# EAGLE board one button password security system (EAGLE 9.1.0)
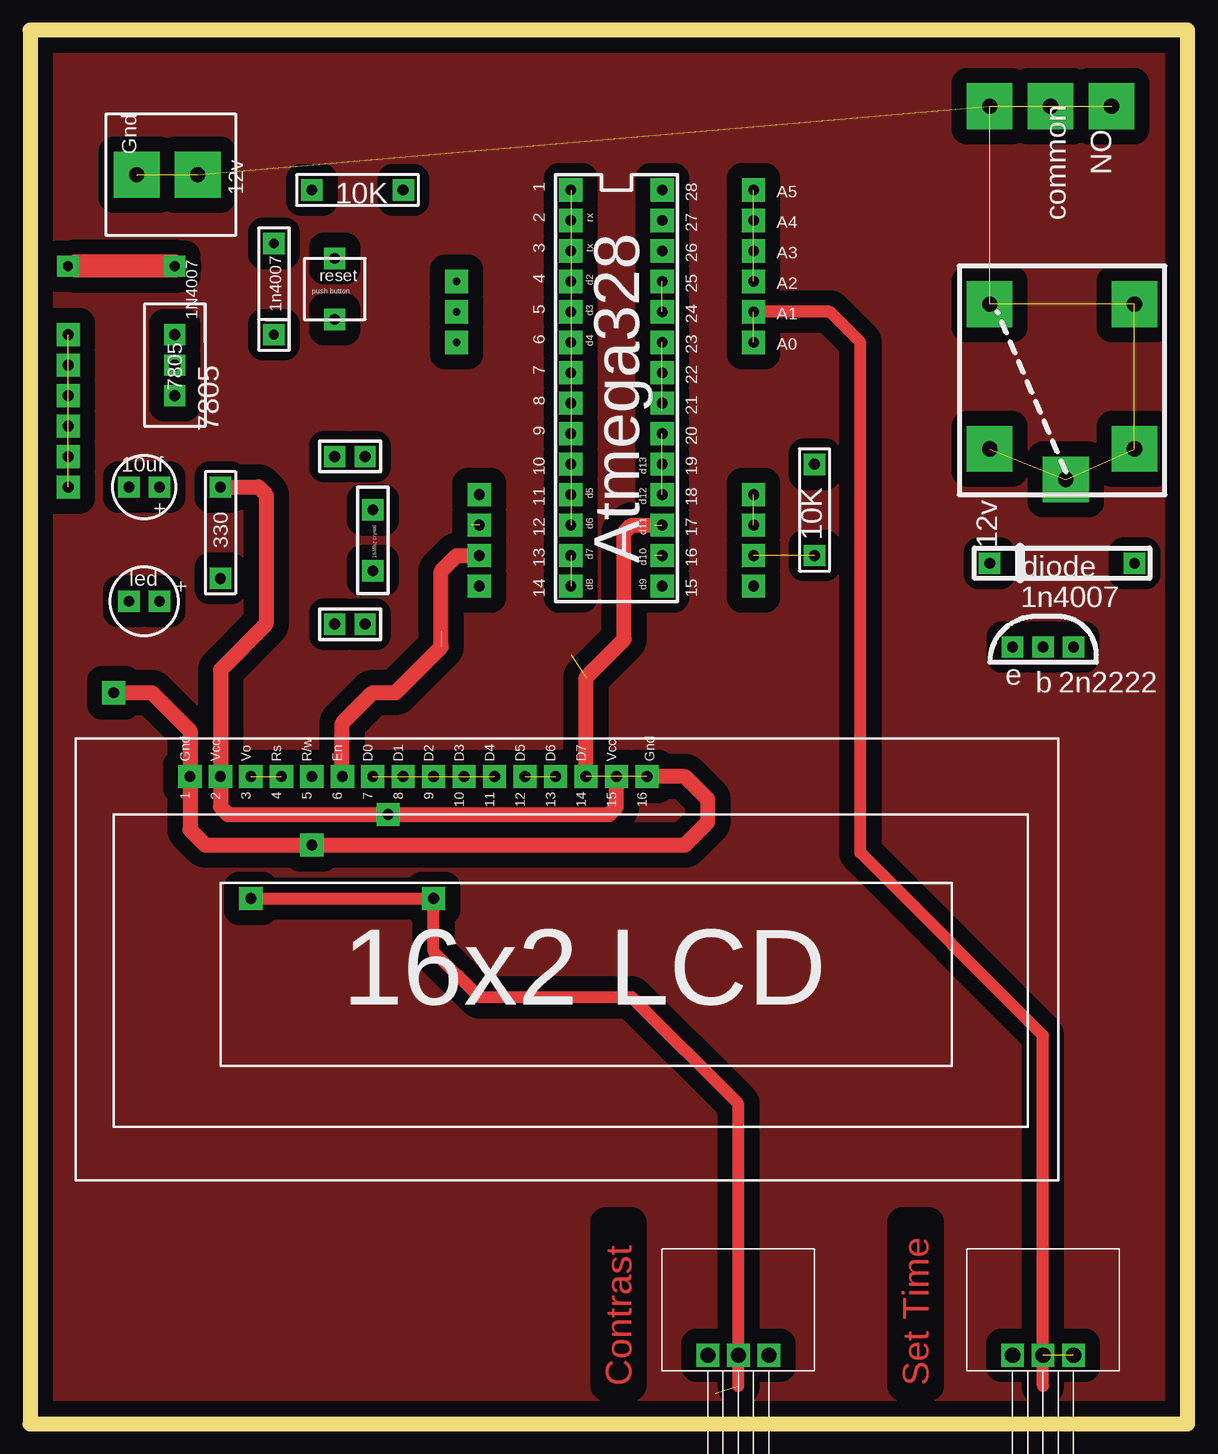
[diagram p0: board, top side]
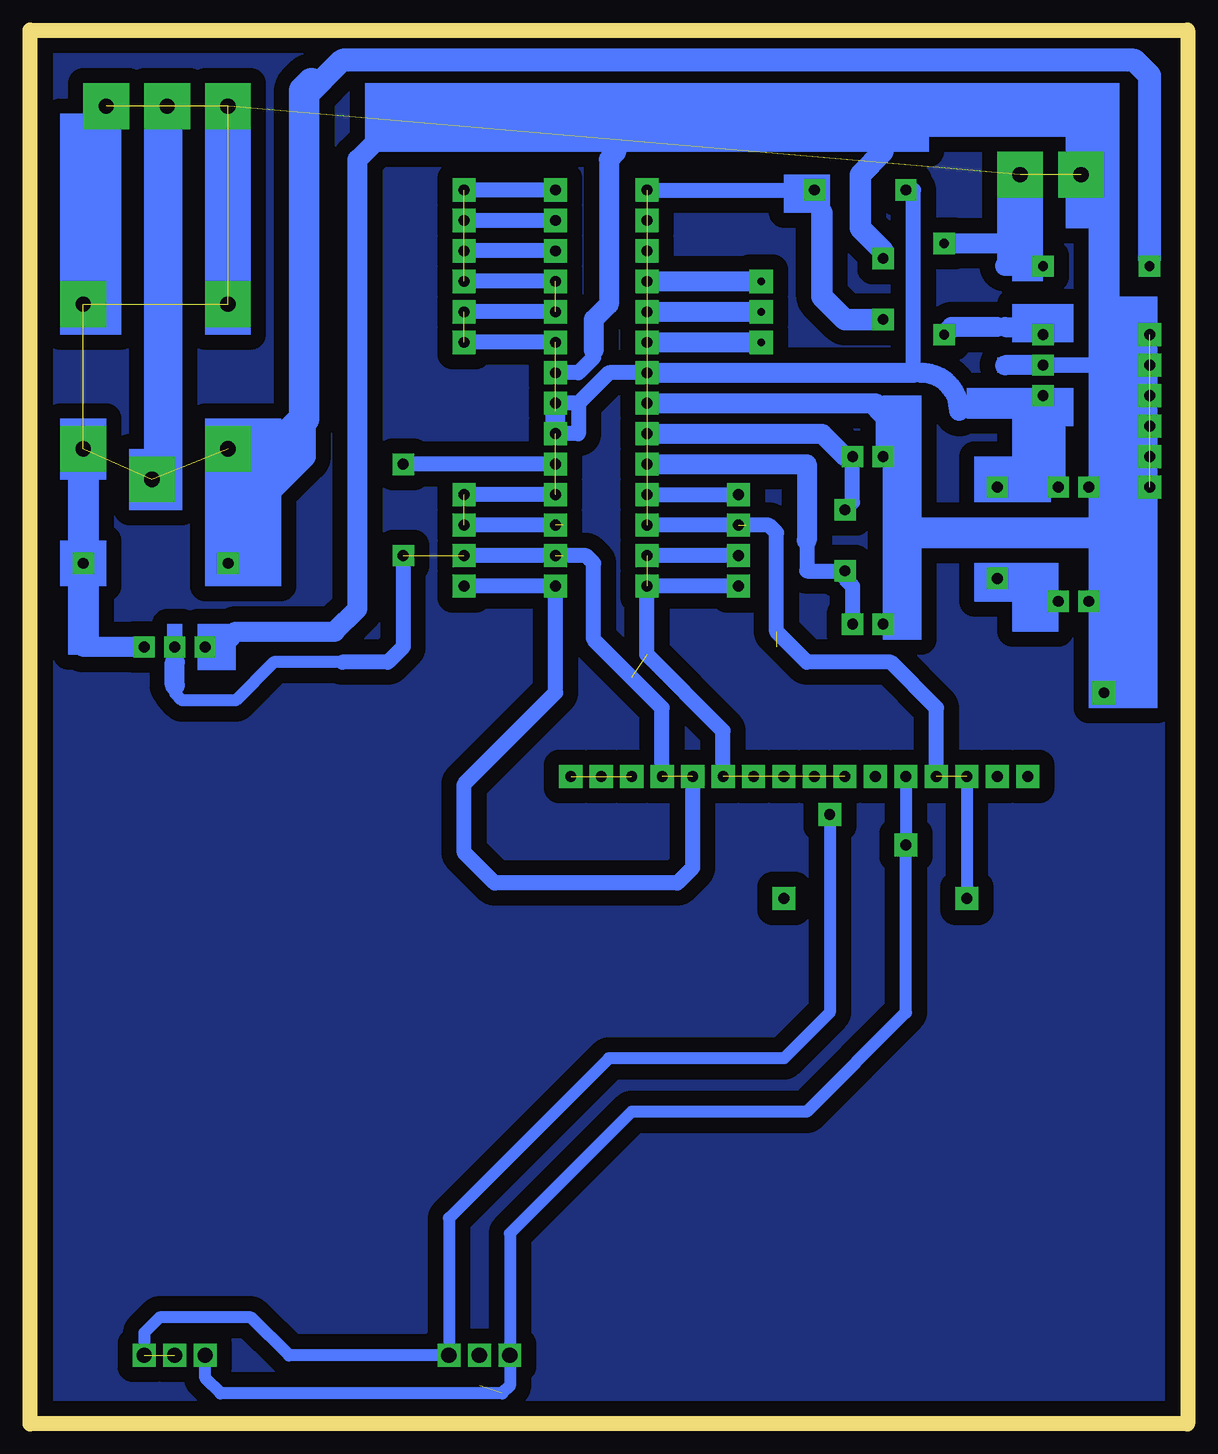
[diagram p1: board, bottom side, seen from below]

Size 96.52 x 116.2 mm. Coordinates in mm from the lower left corner, seen from the top.
Outline: 0,0 96.52,0 96.52,116.2 0,116.2 0,0
Copper layers (1*16): Top 0.035mm / dielectric 1.5mm / Bottom 0.035mm
Design rules "default": minimum track width 10mil, minimum drill 24mil, track to track 8mil, track to pad 8mil, pad to pad 8mil, via to via 8mil, smd to smd 8mil, copper to edge 40mil, drill to drill 8mil, minimum pad ring 10mil, minimum via ring 8mil, stop-mask expansion 4mil, vias tented up to drill 0mil, thermal gap 10mil

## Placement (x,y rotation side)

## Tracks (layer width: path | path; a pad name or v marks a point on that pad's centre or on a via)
1
  pour Bottom (isolate 1.27): 0,116.2 96.52,116.2 96.52,0 0,0
2
  pour Top (isolate 1.27): 0,116.2 96.52,116.2 96.52,0 0,0
S$1  (via drill 0.9 pad 1.78)
  Bottom 1.27: 31.75,73.66 31.75,71.12 v28.57,71.12
  Bottom 1.676: 44.45,80.01 31.75,80.01 31.75,73.66
S$2  (via drill 0.9 pad 1.78, 0.9 pad 1.93, 1.27 pad 1.2)  (40 unrouted)
  Top 1.016: 84.45,3.17 v84.45,5.71 84.45,32.38 69.22,47.62 69.22,90.17 66.67,92.71 v60.33,92.71 | v18.41,43.81 v33.66,43.81 33.66,39.37 37.47,35.56 50.16,35.56 59.05,26.67 v59.05,5.71 59.05,3.17
  Top 1.27: v15.88,78.11 19.05,78.11 19.68,77.47 19.68,66.67 15.88,62.87 v15.88,53.98 15.88,51.44 16.51,50.8 48.26,50.8 48.9,51.44 v48.9,53.98 | v6.99,60.96 10.16,60.96 13.34,57.78 v13.34,53.98 13.34,49.53 14.61,48.26 54.61,48.26 56.52,50.16 56.52,52.07 54.61,53.98 v51.44,53.98 | v26.04,53.98 26.04,58.42 28.57,60.96 30.48,60.96 34.29,64.77 34.29,71.12 35.56,72.39 v37.47,72.39 | v46.35,53.98 46.35,62.23 49.53,65.41 49.53,74.3 50.16,74.93 52.07,74.93
  Bottom 1.016: 81.92,5.71 81.92,3.81 80.64,2.54 57.15,2.54 56.52,3.17 v56.52,5.71 56.52,15.88 46.35,26.04 31.75,26.04 23.5,34.29 v23.5,48.26 v23.5,53.98 | 84.45,61.59 84.45,60.96 83.82,60.33 79.38,60.33 76.2,63.5 70.48,63.5 | v29.84,50.8 29.84,34.29 33.66,30.48 48.26,30.48 61.59,17.14 v61.59,5.71 74.93,5.71 78.11,8.89 85.72,8.89 87,7.62 87,5.71 | v18.41,53.98 v18.41,43.81
  Bottom 1.27: v52.7,80.01 v65.41,80.01 | v65.41,72.39 65.41,64.77 66.67,63.5 70.48,63.5 | v52.7,77.47 v60.33,77.47 | v52.7,74.93 v60.33,74.93 | v52.7,72.39 v60.33,72.39 | v60.33,69.85 v52.7,69.85 52.7,60.96 60.33,53.34 60.33,47.62 57.78,45.09 42.55,45.09 41.27,46.35 v41.27,53.98 | v45.09,77.47 v37.47,77.47 | v37.47,74.93 v45.09,74.93 | v37.47,72.39 v45.09,72.39 | v37.47,69.85 v45.09,69.85 45.09,64.14 38.73,57.78 v38.73,53.98 | v52.7,102.87 v60.33,102.87 | v52.7,100.33 v60.33,100.33 | v52.7,97.79 v60.33,97.79 | v52.7,95.25 v60.33,95.25 | v52.7,92.71 v60.33,92.71 | v52.7,90.17 v60.33,90.17 | v20.95,53.98 20.95,59.69 24.77,63.5 31.75,63.5 34.29,66.04 34.29,74.3 34.92,74.93 36.83,74.93 | v43.81,53.98 43.81,59.69 49.53,65.41 49.53,71.75 50.16,72.39 52.07,72.39
  Bottom 1.676: v52.7,82.55 52.7,84.45 | 84.45,61.59 84.45,63.5
  other vias: 28.57,53.98 31.11,53.98 52.7,87.63 52.7,85.09 45.09,102.87 45.09,100.33 45.09,97.79 45.09,95.25 45.09,92.71 45.09,90.17 45.09,87.63 45.09,85.09 45.09,82.55 45.09,80.01 36.2,53.98 33.66,53.98
S$3
  Bottom 1.676: 80.01,65.41 79.38,66.04 71.12,66.04 69.22,67.94 69.22,105.41 67.31,107.31
S$5  (via drill 0.6 pad 1.93)
  other vias: 35.56,95.25
S$6  (via drill 0.6 pad 1.93)
  other vias: 35.56,92.71
S$7  (via drill 1.27 pad 1.2)
  other vias: 81.92,5.71
S$8  (via drill 0.6 pad 1.93)
  other vias: 35.56,90.17
S$9  (via drill 0.9 pad 1.78)
  other vias: 80.01,93.34
S$10  (via drill 0.9 pad 1.78)
  other vias: 80.01,81.28
S$11  (via drill 0.9 pad 1.78)
  other vias: 80.01,81.28
S$12  (via drill 1.27 pad 1.2)
  other vias: 87,5.71
S$13
  Bottom 1.676: 44.45,95.25 36.2,95.25
S$14
  Bottom 1.676: 44.45,92.71 36.2,92.71
S$15
  Bottom 1.676: 44.45,90.17 36.2,90.17
S$16  (via drill 0.9 pad 1.78)
  other vias: 92.08,81.28
S$17  (via drill 0.9 pad 1.78)
  other vias: 80.01,93.34
S$19  (via drill 0.9 pad 1.78)
  other vias: 80.01,93.34
S$20  (via drill 0.9 pad 1.78)
  other vias: 92.08,93.34
S$21  (via drill 0.9 pad 1.78)
  other vias: 86.36,78.74
S$22  (via drill 0.9 pad 1.78)
  other vias: 80.01,71.75
S$23  (via drill 0.9 pad 1.78)
  other vias: 92.08,71.75
S$24
  Bottom 0.813: 80.01,75.56 80.01,73.66
  Bottom 1.422: 80.01,73.03 80.01,75.56
S$25
  Bottom 1.422: 92.08,73.03 92.08,79.38 92.71,79.38
S$26  (via drill 0.9 pad 1.78)
  other vias: 8.26,78.11
S$27  (via drill 0.9 pad 3.81)  (1 unrouted)
  other vias: 85.09,109.86 80.01,109.86
S$28  (via drill 0.9 pad 3.81)
  other vias: 90.17,109.86
S$29
  Bottom 1.27: 92.08,95.25 90.81,96.52
S$30
  Bottom 1.676: 87.63,64.77 92.08,64.77
S$31  (via drill 0.9 pad 1.93)  (5 unrouted)
  other vias: 3.17,90.81 3.17,88.27 3.17,85.72 3.17,83.19 3.17,80.64 3.17,78.11
S$39  (via drill 1.27 pad 3.81)  (9 unrouted)
  other vias: 92.08,81.28 80.01,81.28 86.36,78.74 92.08,93.34 80.01,93.34 90.17,109.86 85.09,109.86 80.01,109.86 13.97,104.14 8.89,104.14
S$42  (via drill 0.8 pad 1.78)
  Bottom 1.676: v20.32,98.42 15.88,98.42
S$43
  Bottom 1.676: 19.05,84.45 arc-90 22.23,87.63
S$44
  Bottom 1.676: 13.97,96.52 15.24,96.52
S$45
  Bottom 1.676: 15.24,91.44 13.97,91.44
S$48  (via drill 0.8 pad 1.78)
  Top 1.93: v12.06,96.52 3.81,96.52
S$50  (via drill 0.8 pad 1.78)
  other vias: 3.17,96.52
S$51
  Bottom 1.93: 3.17,97.16 3.17,112.39 4.45,113.67 70.48,113.67 73.66,110.49 73.66,83.82 73.66,80.64 76.2,78.11 76.83,78.11
  Bottom 2.54: 73.03,111.76 73.66,111.12 73.66,83.82 74.93,82.55 74.93,80.01
S$65
  Bottom 1.676: 12.7,88.27 15.24,88.27
S$66
  Bottom 1.27: 22.86,88.27 22.86,102.87
S$67  (via drill 0.8 pad 1.78)
  Bottom 1.676: 15.88,91.44 19.68,91.44 v20.32,90.81
S$68
  Bottom 1.27: 13.97,84.45 14.61,85.09
S$69
  Bottom 1.27: 46.99,106.68 47.62,106.05 | 52.07,87.63 50.8,87.63 49.53,88.9 49.53,89.53
  Bottom 1.676: 47.62,106.05 48.26,105.41 48.26,93.34 49.53,92.08 49.53,89.53
S$123  (via drill 0.9 pad 1.78)
  other vias: 81.92,64.77
S$125  (via drill 0.9 pad 1.78)
  other vias: 84.45,64.77
S$126  (via drill 0.9 pad 1.78)
  other vias: 87,64.77
S$319
  Bottom 1.27: 45.09,102.87 33.02,102.87
S$358  (via drill 0.9 pad 1.78)
  other vias: 12.06,90.81
S$359  (via drill 0.9 pad 1.78)
  other vias: 12.06,88.27
S$360  (via drill 0.9 pad 1.78)
  other vias: 12.06,85.72
S$361  (via drill 0.9 pad 1.78)
  Bottom 1.27: v10.79,78.11 10.79,83.82
S$362
  Bottom 1.27: 8.26,88.27 8.89,88.27
S$363  (via drill 0.9 pad 3.81)  (1 unrouted)
  other vias: 13.97,104.14 8.89,104.14
S$365  (via drill 0.9 pad 1.78)
  other vias: 15.88,70.48
S$367  (via drill 0.9 pad 1.78)
  other vias: 10.79,68.58
S$368  (via drill 0.9 pad 1.78)
  other vias: 8.26,68.58
S$392  (via drill 0.9 pad 1.78)
  other vias: 25.4,92.08
S$394  (via drill 0.9 pad 1.78)
  other vias: 25.4,97.16
S$395  (via drill 0.9 pad 1.78)
  other vias: 23.5,102.87
S$396  (via drill 0.9 pad 1.78)
  other vias: 31.11,102.87
S$398
  Bottom 1.778: 26.04,92.08 28.57,92.08 30.48,93.98 30.48,100.97
S$399
  Bottom 1.778: 25.4,97.79 27.3,99.69 27.3,104.14 25.4,106.05
S$401  (via drill 0.9 pad 1.78)
  Bottom 1.27: v28.57,76.2 27.94,76.83 27.94,80.01
S$403  (via drill 0.9 pad 1.78)
  other vias: 25.4,80.64
S$404  (via drill 0.9 pad 1.78)
  other vias: 27.94,80.64
S$405  (via drill 0.9 pad 1.78)
  other vias: 25.4,66.67
S$406  (via drill 0.9 pad 1.78)
  other vias: 27.94,66.67
S$407
  Bottom 1.27: 28.57,70.48 27.94,69.85 27.94,67.31
S$408
  Bottom 1.676: 44.45,82.55 30.48,82.55 28.57,80.64
S$409
  Bottom 1.27: 45.72,87.63 48.26,87.63 50.8,85.09 | 50.8,85.09 52.07,85.09 | 50.8,85.09 50.8,82.55 52.07,82.55
S$412
  Bottom 1.676: 44.45,87.63 22.86,87.63
S$413
  Bottom 1.27: 44.45,85.09 26.67,85.09 25.4,83.82 25.4,81.28
  Bottom 1.676: 44.45,85.09 26.04,85.09
(copper drawn outside any net)
  shapes: Bottom area x51

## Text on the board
Top: Contrast | Set Time
tPlace: Gnd | 12v | 10K | 1 | 28 | NO | A5 | 2 | rx | 27 | A4 | common | 3 | tx | 26 | A3 | 4 | d2 | 25 | reset | push button | A2 | 1n4007 | 5 | d3 | 24 | 1N4007 | A1 | 6 | d4 | 23 | 7805 | A0 | 7805 | 7 | 22 | 8 | 21 | 9 | 20 | 10 | d13 | 19 | 10uf | 11 | d5 | d12 | 18 | + | 12 | d6 | d11 | 17 | 16Mhz crystal | 10K | 330 | 13 | d7 | d10 | 16 | 12v | Atmega328 | diode | led | 14 | d8 | d9 | 15 | 1n4007 | + | e | b | 2n2222 | Gnd | Vcc | Vo | Rs | R/w | En | D0 | D1 | D2 | D3 | D4 | D5 | D6 | D7 | Vcc | Gnd | 1 | 2 | 3 | 4 | 5 | 6 | 7 | 8 | 9 | 10 | 11 | 12 | 13 | 14 | 15 | 16 | 16x2 LCD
